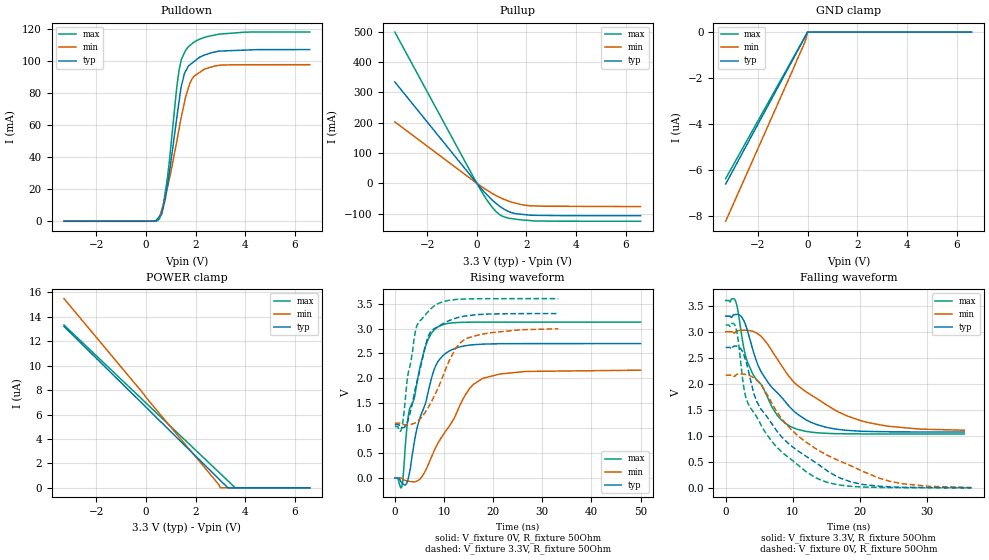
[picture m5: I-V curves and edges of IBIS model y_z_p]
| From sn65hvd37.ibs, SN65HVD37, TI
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|   y_z Model
[Model]   y_z_p
Model_type   3-state
Polarity   Non-Inverting
Vmeas = 1.65
Vref = 1.65
Cref = 50pF
Rref = 50
|   typ   min   max
|   (nom PVT)   (fast PVT)   (slow PVT)
|C_Comp from frequency method(F=10MHz)
|C_comp   8.746e-11   8.667e-11   1.110e-10
|ON state
|C_comp   8.746e-11   8.667e-11   1.110e-10
|OFF state
|C_comp   1.822e-11   1.815e-11   1.847e-11
|C_Comp from L-C Tank method(L=1nH)
|Resonant Frequency(Hz)   1.320e+09   1.360e+09   1.280e+09
C_comp   1.455e-11   1.371e-11   1.548e-11
|ON state
|Resonant Frequency(Hz)   1.320e+09   1.360e+09   1.280e+09
|C_comp   1.455e-11   1.371e-11   1.548e-11
|OFF state
|Resonant Frequency(Hz)   1.490e+09   1.540e+09   1.450e+09
|C_comp   1.142e-11   1.069e-11   1.206e-11
| Where nom  PVT is Nominal Process, 3.3V, 27C
|   Fast PVT is Strong Process,  3.6V, -40C
|   Slow PVT is Weak Process,   3V, 125C
[Voltage Range]   3.3   3   3.6
|Ambient Temperature   25   85   -40
|Junction Temperature
[Temperature Range]   27   125   -40
[Pullup Reference]   3.3   3   3.6
[Pulldown Reference]   0   0   0
[Power Clamp Reference]   3.3   3   3.6
[GND Clamp Reference]   0   0   0
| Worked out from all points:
|   slope of the pulldown table from 0 to 0.495 V, typ, clamps not added: 253 ohm
|   slope of the pullup table from 0 to 0.495 V, typ, clamps not added: 11 ohm
|   falling waveform, V_fixture 3.3V, R_fixture 50Ohm: 20-80 % time 6.21ns typ, 9.43ns min, 4.72ns max; typ from 3.3 V to 1.07 V
|   rising waveform, V_fixture 0V, R_fixture 50Ohm: 20-80 % time 4.27ns typ, 7.26ns min, 3.72ns max; typ from 0 V to 2.7 V
|   rising waveform, V_fixture 3.3V, R_fixture 50Ohm: 20-80 % time 3.27ns typ, 5.35ns min, 2.51ns max; typ from 1.07 V to 3.3 V
|   falling waveform, V_fixture 0V, R_fixture 50Ohm: 20-80 % time 9.18ns typ, 11.9ns min, 6.77ns max; typ from 2.7 V to 0.003 V
[Pulldown]
|   Voltage   I(typ)   I(min)   I(max)
-3.3V     -1.596nA   -10.33nA   -384.2pA
326.7mV   33.39uA    104.4uA    55.43uA
540mV     2.779mA    2.8mA      1.538mA
633.6mV   4.495mA    6.841mA    5.548mA
860.4mV   21.76mA    20.65mA    26.43mA
1.242V    64.5mA     49.71mA    83.62mA
1.332V    74.42mA    57.38mA    94mA
1.554V    92.36mA    74.35mA    105.1mA
1.761V    97.45mA    85.72mA    109.5mA
1.912V    99.29mA    89.91mA    111.5mA
3.074V    106.2mA    97.52mA    116.9mA
6.6V      107.1mA    97.67mA    118mA
[GND Clamp]
|   Voltage   I(typ)   I(min)   I(max)
-3.3V     -6.611uA   -8.231uA   -6.374uA
-171mV    -350.3nA   -590.2nA   -330.9nA
-69mV     -145.4nA   -310.2nA   -134nA
-24mV     -52.22nA   -125nA     -46.97nA
-3.3mV    0A         0A         0A
6.6V      0A         0A         0A
[Pullup]
|   Voltage   I(typ)   I(min)   I(max)
-3.3V     333.9mA    202.1mA    498.5mA
82.8mV    -8.117mA   -4.816mA   -12.03mA
478.8mV   -43.63mA   -26.58mA   -63.63mA
648mV     -57.42mA   -35.04mA   -81.84mA
885.6mV   -73.74mA   -45.37mA   -101.5mA
1.062V    -83.72mA   -52.1mA    -110.1mA
1.403V    -97.21mA   -62.39mA   -116.8mA
1.836V    -102.9mA   -71.53mA   -121.2mA
2.168V    -105.7mA   -74.55mA   -123.3mA
6.6V      -107.2mA   -77.14mA   -125.6mA
[POWER Clamp]
|   Voltage   I(typ)   I(min)   I(max)
-3.3V     13.22uA    15.49uA    13.33uA
2.844V    915.9nA    494nA      1.459uA
3V        603.9nA    0A         1.158uA
3.297V    0A         0A         585.2nA
3.596V    0A         0A         0A
6.6V      0A         0A         0A
[Ramp]
R_load = 50
|   typ   min   max
dV/dt_r   1.61828/4.26467e-09   1.29837/7.23985e-09   1.87722/3.71913e-09
dV/dt_f   1.33667/6.21964e-09   1.13863/9.49493e-09   1.53953/4.72472e-09
[Falling Waveform]
V_fixture = 3.3V
V_fixture_min = 3V
V_fixture_max = 3.6V
R_fixture = 50Ohm
|   Time   V(typ)   V(min)   V(max)
0s        3.3V       3V         3.6V
1.5ns     3.331V     2.999V     3.58V
2.44ns    3.273V     3.029V     2.881V
3.29ns    2.999V     3.029V     2.404V
5.23ns    2.243V     2.915V     1.995V
7.67ns    1.83V      2.477V     1.395V
9.53ns    1.555V     2.126V     1.187V
13.67ns   1.211V     1.707V     1.059V
19.99ns   1.09V      1.296V     1.037V
35.5ns    1.073V     1.108V     1.034V
[Rising Waveform]
V_fixture = 0V
V_fixture_min = 0V
V_fixture_max = 0V
R_fixture = 50Ohm
|   Time   V(typ)   V(min)   V(max)
0s        25.24nV    80.6nV     25.61nV
1.43ns    -95.6mV    -9.065mV   -168.1mV
2.47ns    -97.05mV   -58.21mV   1.026V
2.93ns    77.16mV    -66.74mV   1.357V
4.57ns    1.021V     -58.48mV   1.951V
6.18ns    1.479V     136.8mV    2.619V
8.71ns    2.326V     687.9mV    3.028V
15.21ns   2.666V     1.794V     3.127V
18.13ns   2.687V     2.007V     3.128V
50ns      2.697V     2.164V     3.129V
[Rising Waveform]
V_fixture = 3.3V
V_fixture_min = 3V
V_fixture_max = 3.6V
R_fixture = 50Ohm
|   Time   V(typ)   V(min)   V(max)
0s        1.071V     1.101V     1.032V
1.43ns    1.009V     1.089V     1.01V
2.61ns    1.138V     1.069V     2.033V
4.5ns     1.928V     1.129V     3.062V
6.58ns    2.78V      1.379V     3.317V
7.9ns     2.988V     1.618V     3.444V
12.11ns   3.199V     2.555V     3.579V
14.13ns   3.247V     2.772V     3.592V
19.53ns   3.291V     2.916V     3.599V
33.26ns   3.3V       2.995V     3.6V
[Falling Waveform]
V_fixture = 0V
V_fixture_min = 0V
V_fixture_max = 0V
R_fixture = 50Ohm
|   Time   V(typ)   V(min)   V(max)
0s        2.698V     2.165V     3.13V
1.52ns    2.725V     2.169V     3.074V
2.77ns    2.533V     2.183V     1.867V
3.37ns    2.257V     2.166V     1.612V
5.22ns    1.521V     1.985V     1.22V
8.26ns    989.9mV    1.343V     700.8mV
12.03ns   601.1mV    874.1mV    305.3mV
20.15ns   72.16mV    333.5mV    18.76mV
26.16ns   13.49mV    82.19mV    4.748mV
36.56ns   2.857mV    9.151mV    1.512mV
